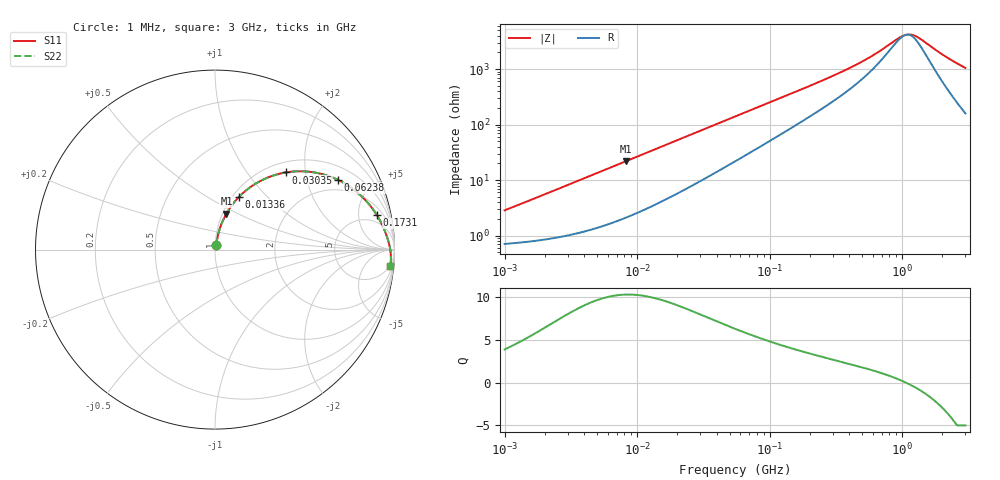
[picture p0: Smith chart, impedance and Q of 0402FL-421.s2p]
# MHz S MA R 50
!Freq  MagS11  AngS11  MagS21  AngS21  MagS12  AngS12  MagS22  AngS22
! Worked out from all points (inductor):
!   801 points, 1 MHz to 3 GHz, reference 50 ohm
!   read as one part in series: L = 439 nH near 1.041 MHz
!   highest Q = 10.3 at 8.262 MHz (marker M1), where L = 422 nH
!   self-resonance near 1.074 GHz
!   S11 on the Smith chart (normalised r, x): 1 MHz: 1.01, +0.06; 13.36 MHz: 1.07, +0.70; 30.35 MHz: 1.20, +1.55; 62.38 MHz: 1.52, +3.12; 173.1 MHz: 3.24, +8.30; 3 GHz: 4, -21
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1  0.02842 74.1  0.9926 -1.6  0.9926 -1.6  0.02842 74.1
3.823119  0.1021 77.8  0.9835 -5.8  0.9835 -5.8  0.1021 77.8
8.262105  0.2107 72.4  0.9575 -12.1  0.9575 -12.1  0.2107 72.4
13.35728  0.3219 65.6  0.9151 -18.7  0.9151 -18.7  0.3219 65.6
14.47069  0.3441 64.2  0.9047 -20.0  0.9047 -20.0  0.3441 64.2
20.74721  0.4549 56.8  0.8417 -26.9  0.8417 -26.9  0.4549 56.8
30.3475  0.5823 47.5  0.7436 -35.3  0.7436 -35.3  0.5823 47.5
40.5666  0.6752 40.1  0.6499 -42.0  0.6499 -42.0  0.6752 40.1
54.77226  0.7579 32.5  0.5446 -48.5  0.5446 -48.5  0.7579 32.5
62.38265  0.7882 29.5  0.499 -51.0  0.499 -51.0  0.7882 29.5
100.8535  0.871 19.8  0.3452 -58.5  0.3452 -58.5  0.871 19.8
173.1398  0.9223 12.0  0.2146 -62.9  0.2146 -62.9  0.9223 12.0
209.4008  0.9337 9.9  0.1795 -63.5  0.1795 -63.5  0.9337 9.9
457.0858  0.962 4.0  0.0786 -59.1  0.0786 -59.1  0.962 4.0
604.9187  0.9679 2.6  0.05438 -52.6  0.05438 -52.6  0.9679 2.6
792.5923  0.9725 1.3  0.0356 -38.7  0.0356 -38.7  0.9725 1.3
1017.911  0.9759 0.2  0.02445 -9.2  0.02445 -9.2  0.9759 0.2
1113.852  0.9769 -0.2  0.02325 6.6  0.02325 6.6  0.9769 -0.2
1206.698  0.9778 -0.5  0.02387 21.1  0.02387 21.1  0.9778 -0.5
1374.365  0.979 -1.1  0.02803 41.0  0.02803 41.0  0.979 -1.1
2199.798  0.9817 -3.4  0.06138 71.0  0.06138 71.0  0.9817 -3.4
3000  0.9816 -5.3  0.0935 76.0  0.0935 76.0  0.9816 -5.3
